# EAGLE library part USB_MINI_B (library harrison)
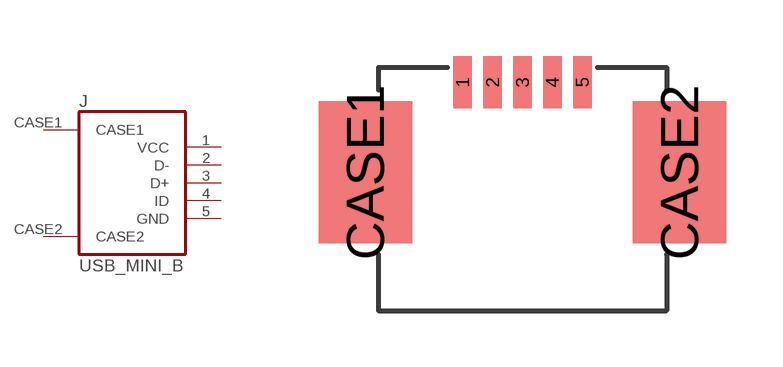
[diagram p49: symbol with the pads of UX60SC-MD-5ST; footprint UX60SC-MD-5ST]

Designator prefix J

## USB_MINI_B  [UX60SC-MD-5ST]
1  VCC  pwr
2  D-
3  D+
4  ID  in
5  GND  pwr
CASE1  CASE1  pas
CASE2  CASE2  pas

## Footprint UX60SC-MD-5ST (pad centres in mm)
smd 0.5 x 1.4: 1 -1.6,2.6; 2 -0.8,2.6; 3 0,2.6; 4 0.8,2.6; 5 1.6,2.6
smd 2.5 x 3.8: CASE1 -4.2,0.2; CASE2 4.2,0.2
